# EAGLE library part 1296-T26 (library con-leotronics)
1.27mm SINGLE ROW FEMALE SOCKET Source: http://www.leotronics.co.uk/Conexcon/Data%20Sheets/sec.%20A/1296ing.pdf
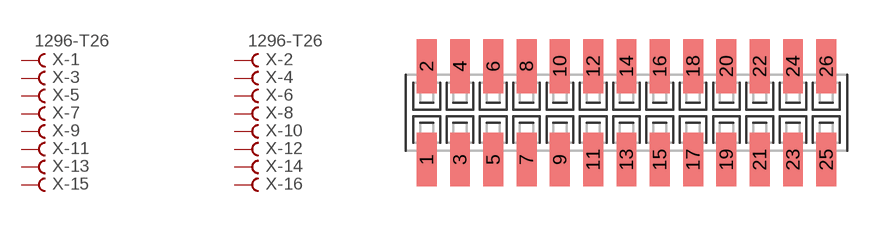
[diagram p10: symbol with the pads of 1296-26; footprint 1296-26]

Designator prefix X; gates -1=FVAL -2=FVAL -3=F -4=F -5=F -6=F -7=F -8=F -9=F -10=F -11=F -12=F -13=F -14=F -15=F -16=F -17=F -18=F -19=F -20=F -21=F -22=F -23=F -24=F -25=F -26=F

## 1296-T26 (OC_FARNELL: unknown; OC_NEWARK: unknown)  [1296-26]
1  -1:B  pas
2  -2:B  pas
3  -3:B  pas
4  -4:B  pas
5  -5:B  pas
6  -6:B  pas
7  -7:B  pas
8  -8:B  pas
9  -9:B  pas
10  -10:B  pas
11  -11:B  pas
12  -12:B  pas
13  -13:B  pas
14  -14:B  pas
15  -15:B  pas
16  -16:B  pas
17  -17:B  pas
18  -18:B  pas
19  -19:B  pas
20  -20:B  pas
21  -21:B  pas
22  -22:B  pas
23  -23:B  pas
24  -24:B  pas
25  -25:B  pas
26  -26:B  pas

## Footprint 1296-26 (pad centres in mm)
1.27mm SINGLE ROW FEMALE SOCKET Source: http://www.leotronics.co.uk/Conexcon/Data%20Sheets/sec.%20A/1296ing.pdf
smd 0.76 x 2.05: 1 -7.62,-1.78; 2 -7.62,1.78; 3 -6.35,-1.78; 4 -6.35,1.78; 5 -5.08,-1.78; 6 -5.08,1.78; 7 -3.81,-1.78; 8 -3.81,1.78; 9 -2.54,-1.78; 10 -2.54,1.78; 11 -1.27,-1.78; 12 -1.27,1.78; 13 0,-1.78; 14 0,1.78; 15 1.27,-1.78; 16 1.27,1.78; 17 2.54,-1.78; 18 2.54,1.78; 19 3.81,-1.78; 20 3.81,1.78; 21 5.08,-1.78; 22 5.08,1.78; 23 6.35,-1.78; 24 6.35,1.78; 25 7.62,-1.78; 26 7.62,1.78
